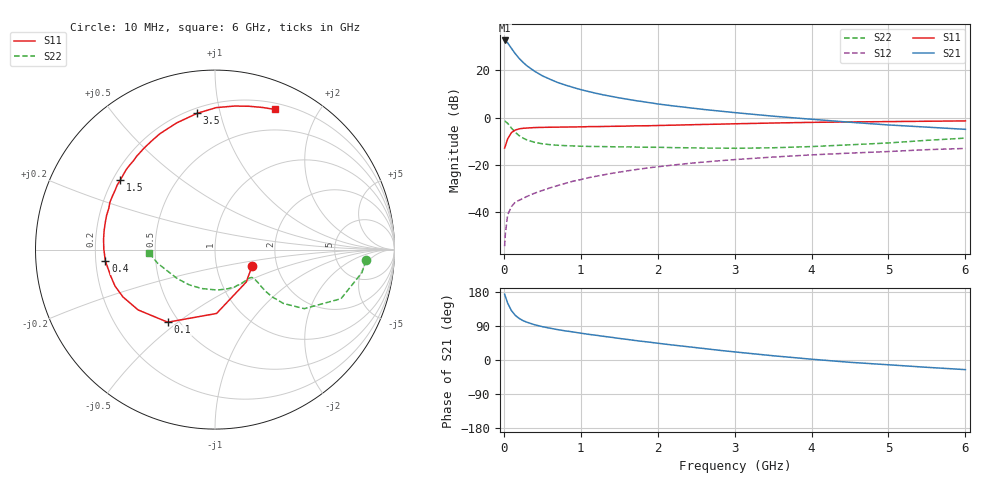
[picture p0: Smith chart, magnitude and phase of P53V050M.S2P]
! SIEMENS Small Signal Semiconductors
! BFP183
! Si NPN RF Bipolar Junction Transistor in SOT143
! VCE = 3 V  IC = 50 mA
! Common Emitter S-Parameters:  March  1996
# GHz  S  MA  R  50
!  f  S11  S21  S12  S22
! GHz  MAG  ANG  MAG  ANG  MAG  ANG  MAG  ANG
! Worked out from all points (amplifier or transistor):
!   36 points, 10 MHz to 6 GHz, reference 50 ohm
!   highest |S21| = 32.6 dB at 10 MHz (marker M1)
!   |S21| within 3 dB of that: start of sweep to 91.6 MHz
!   unconditionally stable (mu >= 1): start of sweep to 19.32 MHz; 300.1 MHz to end of sweep
!   at 250 MHz: K = 0.91, MSG = 28.8 dB, |S12| = -34.2 dB
!   at 1.4 GHz: K = 1.41, MAG = 12.5 dB, |S12| = -23.6 dB
!   at 6 GHz: K = 1.09, MAG = 2.2 dB, |S12| = -13.1 dB
!   S11 on the Smith chart (normalised r, x): 10 MHz: 1.49, -0.29; 100 MHz: 0.44, -0.46; 400 MHz: 0.24, -0.05; 1.5 GHz: 0.23, +0.31; 3.5 GHz: 0.23, +0.85; 6 GHz: 0.26, +1.48
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0.01  0.2261 -24.0  42.75 173.6  0.0019 68.0  0.8428 -4.1
0.02  0.251 -46.1  42.29 167.4  0.0035 75.4  0.8285 -8.9
0.05  0.3559 -88.6  38.03 150.0  0.0088 69.8  0.7534 -21.3
0.1  0.4828 -123.1  28.9 130.0  0.0131 53.8  0.5963 -33.5
0.15  0.5446 -141.9  22.27 117.6  0.0164 51.0  0.4849 -38.2
0.2  0.5764 -152.7  17.77 109.6  0.0178 50.2  0.4125 -39.6
0.25  0.5931 -160.0  14.68 103.8  0.0194 50.6  0.3675 -39.5
0.3  0.5997 -165.9  12.44 99.7  0.0214 51.5  0.3355 -38.8
0.4  0.6141 -174.1  9.527 93.0  0.0251 55.2  0.2993 -37.4
0.5  0.6196 179.7  7.655 88.0  0.0286 56.3  0.2785 -36.8
0.6  0.6236 174.6  6.464 83.9  0.0325 58.4  0.2671 -36.6
0.7  0.627 170.0  5.513 80.2  0.0364 60.4  0.2593 -37.0
0.9  0.6333 162.7  4.342 74.0  0.045 60.8  0.2507 -38.9
1.1  0.6421 155.7  3.556 67.8  0.0534 60.9  0.245 -41.8
1.5  0.6543 143.8  2.61 56.9  0.07 59.2  0.24 -49.4
1.8  0.6692 135.1  2.176 49.2  0.0827 57.3  0.2358 -56.7
2.2  0.6897 125.0  1.765 39.4  0.0989 53.7  0.2309 -67.1
2.8  0.7245 111.0  1.374 25.6  0.1216 47.7  0.2258 -85.3
3.5  0.766 97.4  1.069 11.2  0.1459 41.1  0.2294 -108.9
4.5  0.8071 82.3  0.796 -6.1  0.1768 31.1  0.265 -142.3
5.5  0.8347 71.6  0.627 -19.3  0.2092 22.3  0.3297 -166.9
6  0.8493 66.9  0.563 -25.4  0.222 17.2  0.3673 -177.2
